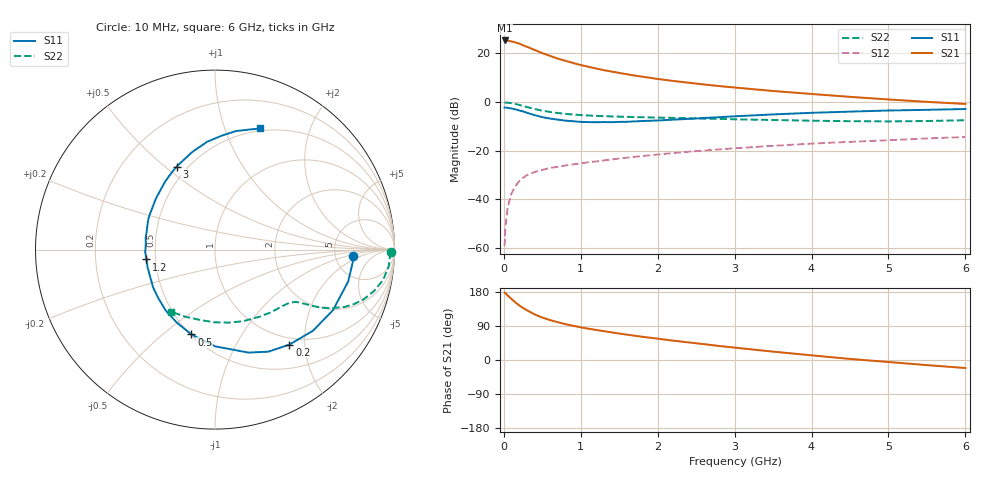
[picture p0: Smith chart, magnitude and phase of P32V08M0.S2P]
! SIEMENS Small Signal Semiconductors
! BFP181
! Si NPN RF Bipolar Junction Transistor in SOT143
! VCE = 2 V  IC = 8 mA
! Common Emitter S-Parameters:  March  1996
# GHz  S  MA  R  50
!  f  S11  S21  S12  S22
! GHz  MAG  ANG  MAG  ANG  MAG  ANG  MAG  ANG
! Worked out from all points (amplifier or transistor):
!   36 points, 10 MHz to 6 GHz, reference 50 ohm
!   highest |S21| = 25.3 dB at 10 MHz (marker M1)
!   |S21| within 3 dB of that: start of sweep to 331.3 MHz
!   unconditionally stable (mu >= 1): 1.161 GHz to end of sweep
!   at 250 MHz: K = 0.31, MSG = 27.2 dB, |S12| = -31.1 dB
!   at 1.4 GHz: K = 1.08, MAG = 16.3 dB, |S12| = -23.6 dB
!   at 6 GHz: K = 1.03, MAG = 5.7 dB, |S12| = -14.3 dB
!   S11 on the Smith chart (normalised r, x): 10 MHz: 7.44, -1.38; 200 MHz: 0.88, -1.70; 500 MHz: 0.51, -0.63; 1.2 GHz: 0.45, -0.06; 3 GHz: 0.44, +0.55; 6 GHz: 0.47, +1.33
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0.01  0.7702 -2.8  18.41 178.0  0.0011 83.4  0.9805 -0.8
0.02  0.7703 -5.5  18.41 176.4  0.0027 90.3  0.9756 -2.0
0.05  0.763 -13.5  18.32 170.2  0.007 85.6  0.973 -5.3
0.1  0.7388 -27.2  17.56 161.0  0.0133 74.7  0.9516 -10.3
0.15  0.7086 -39.7  16.79 152.0  0.0188 69.9  0.9143 -14.7
0.2  0.6724 -51.9  15.86 144.1  0.0239 65.0  0.8737 -18.5
0.25  0.6421 -62.3  14.64 137.2  0.0278 61.4  0.8303 -21.5
0.3  0.6034 -72.0  13.66 131.3  0.0316 57.8  0.7909 -23.8
0.4  0.539 -89.9  11.76 120.3  0.0366 53.1  0.7201 -27.0
0.5  0.4906 -105.5  10.1 112.0  0.0405 49.8  0.6664 -28.9
0.6  0.4589 -117.7  8.898 105.4  0.0444 48.3  0.627 -30.0
0.7  0.4363 -129.1  7.808 99.8  0.0469 47.3  0.5967 -30.8
0.8  0.4155 -139.6  7.031 94.7  0.0499 46.1  0.5731 -31.5
1.1  0.3884 -165.2  5.306 82.5  0.0582 46.0  0.5302 -33.4
1.2  0.3856 -171.8  4.888 79.3  0.0605 45.6  0.5217 -34.3
1.7  0.4012 159.6  3.503 64.1  0.075 45.5  0.4929 -39.3
2.2  0.4353 139.2  2.717 51.1  0.0897 43.8  0.4732 -45.9
3  0.5098 114.8  1.989 32.7  0.1125 39.6  0.4428 -58.8
3.5  0.558 103.2  1.689 22.1  0.1265 36.6  0.4289 -68.4
4.5  0.6366 86.5  1.28 2.8  0.1525 29.2  0.4051 -90.4
5.5  0.6932 74.5  1.01 -13.5  0.1791 22.5  0.4089 -113.7
6  0.7201 69.6  0.915 -21.2  0.1921 18.4  0.4233 -125.4
